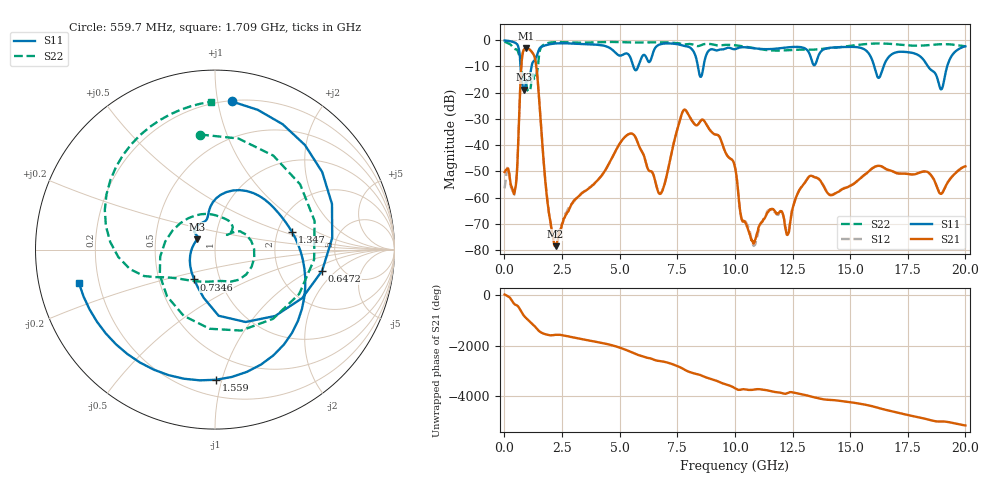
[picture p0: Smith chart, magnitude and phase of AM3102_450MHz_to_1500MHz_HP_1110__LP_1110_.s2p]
!Agilent Technologies,E8364B,MY43040894,A.07.50.67
!Agilent E8364B: A.07.50.67
!Date: Thursday, January 11, 2018 06:47:43
!Correction: S11(Full 2 Port(1,2))
!S21(Full 2 Port(1,2))
!S12(Full 2 Port(1,2))
!S22(Full 2 Port(1,2))
!S2P File: Measurements: S11, S21, S12, S22:
# Hz S  dB  R 50
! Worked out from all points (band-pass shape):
!   1601 points, 10 MHz to 20 GHz, reference 50 ohm
!   highest |S21| = -3.15 dB at 959.5 MHz (marker M1); lowest = -78.5 dB at 2.221 GHz (marker M2)
!   |S21| within 3 dB of the highest: 773.4 MHz to 1.302 GHz (528.7 MHz wide, 50.9 % of centre)
!   lowest |S11| = -18.8 dB at 859.6 MHz (marker M3), VSWR 1.26, Z = 40.7 + j4.74 ohm
!   |S11| at or under -10 dB: 703.8 MHz to 1.178 GHz (473.8 MHz wide, 50.4 % of centre); 16.05 GHz to 16.45 GHz (401.6 MHz wide, 2.47 % of centre); 18.38 GHz to 19.21 GHz (831.6 MHz wide, 4.42 % of centre)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
!   |S22| runs from -19.6 to -0.5 dB; largest |S21 - S12| = 0.0017
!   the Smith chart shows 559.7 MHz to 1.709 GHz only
!   S11 on the Smith chart (normalised r, x): 559.7 MHz: 0.21, +1.10; 647.2 MHz: 3.57, -1.34; 734.6 MHz: 0.75, -0.26; 1.347 GHz: 2.41, +0.58; 1.559 GHz: 0.31, -0.96; 1.709 GHz: 0.12, -0.12
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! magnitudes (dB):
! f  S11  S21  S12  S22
! 10 MHz  -0.1  -50.2  -56.5  -0.5
! 409.8 MHz  -0.8  -58.6  -59.2  -3.2
! 559.7 MHz  -1.6  -47.9  -47.7  -3.8
! 647.2 MHz  -4.3  -27.3  -27.2  -6.0
! 734.6 MHz  -13.9  -10.0  -10.0  -11.0
! 859.6 MHz  -18.8  -3.4  -3.5  -14.6
! 959.5 MHz  -15.6  -3.1  -3.2  -17.1
! 1.347 GHz  -7.1  -7.7  -7.7  -14.6
! 1.559 GHz  -2.8  -29.1  -29.1  -3.4
! 1.709 GHz  -2.1  -46.8  -46.7  -1.7
! 2.221 GHz  -1.2  -78.5  -75.1  -0.7
! 3.346 GHz  -1.4  -58.4  -58.3  -0.9
! 5.482 GHz  -6.9  -35.5  -35.6  -0.8
! 6.682 GHz  -1.8  -57.9  -58.0  -0.8
! 7.806 GHz  -2.2  -26.5  -26.5  -1.6
! 10.01 GHz  -3.4  -48.4  -48.3  -1.9
! 10.82 GHz  -3.1  -77.4  -78.4  -3.0
! 12.29 GHz  -2.7  -74.1  -73.7  -3.8
! 13.34 GHz  -7.9  -51.7  -51.7  -3.6
! 16.68 GHz  -6.4  -49.5  -49.5  -1.4
! 18.95 GHz  -18.7  -58.5  -58.3  -1.5
! 20 GHz  -2.3  -48.0  -48.0  -2.3
